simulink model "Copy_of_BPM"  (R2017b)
settings: Solver=FixedStepDiscrete  StartTime=0.0  StopTime=10.0  FixedStep=0.01  RelTol=1e-3  EnableMultiTasking=on
undefined symbols (not defined in the file): ASWTYPE_FALSE, CcBPM_KL30CHiVolt_mV, CcBPM_KL30CLoVolt_mV, CcBPM_KL30CTooHiVolt_mV, CcBPM_KL30CTooLoVolt_mV, CcBPM_KL30CVoltRtnDifVal_mV, CcBPM_KL30HiVolt_mV, CcBPM_KL30LoVolt_mV, CcBPM_KL30TooHiVolt_mV, CcBPM_KL30TooLoVolt_mV, CcBPM_KL30VoltRtnDifVal_mV, Enum_ISPBMULastPwrDown, Enum_ISPBMULastReset, Enum_ISPDiagComSt, Enum_ISPNetWkUpSt, Enum_MSMBMUState
libraries: AIWAYS_Powertrain_BMS_lib x15

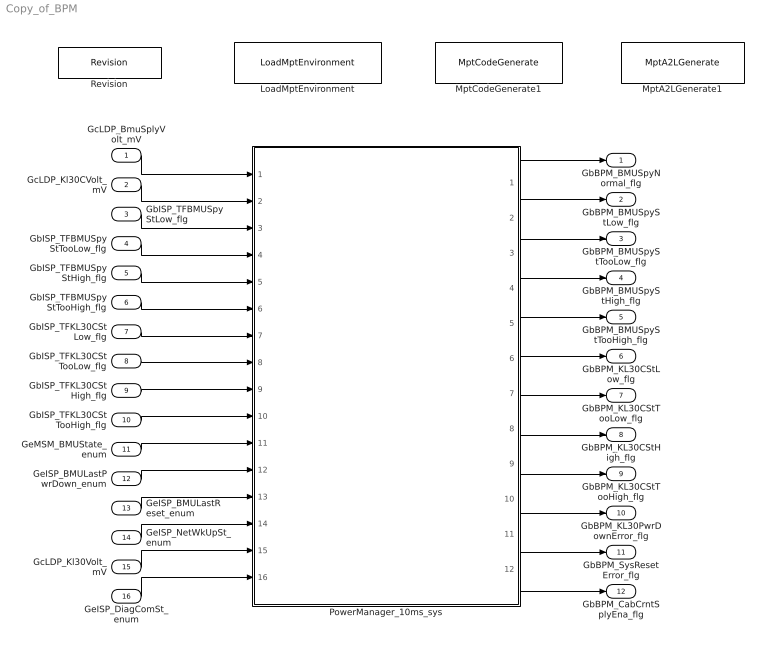
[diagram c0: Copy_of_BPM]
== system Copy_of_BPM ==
  GcLDP_BmuSplyVolt_mV : Inport
  GcLDP_Kl30CVolt_mV : Inport  Port=2
  GbISP_TFBMUSpyStLow_flg : Inport  Port=3
  GbISP_TFBMUSpyStTooLow_flg : Inport  Port=4
  GbISP_TFBMUSpyStHigh_flg : Inport  Port=5
  GbISP_TFBMUSpyStTooHigh_flg : Inport  Port=6
  GbISP_TFKL30CStLow_flg : Inport  Port=7
  GbISP_TFKL30CStTooLow_flg : Inport  Port=8
  GbISP_TFKL30CStHigh_flg : Inport  Port=9
  GbISP_TFKL30CStTooHigh_flg : Inport  Port=10
  GeMSM_BMUState_enum : Inport  Port=11
  GeISP_BMULastPwrDown_enum : Inport  Port=12
  GeISP_BMULastReset_enum : Inport  Port=13
  GeISP_NetWkUpSt_enum : Inport  Port=14
  GcLDP_Kl30Volt_mV : Inport  Port=15
  GeISP_DiagComSt_enum : Inport  Port=16
  LoadMptEnvironment : AIWAYS_Powertrain_BMS_lib/Config/LoadMptEnvironment  ProjectName=Comm  SuppierID=NewPlatformUAES
  MptA2LGenerate1 : AIWAYS_Powertrain_BMS_lib/Config/MptA2LGenerate  SystemSampleTime=-1
  MptCodeGenerate1 : AIWAYS_Powertrain_BMS_lib/Config/MptCodeGenerate  SystemSampleTime=-1
  PowerManager_10ms_sys : Subsystem
  Revision : AIWAYS_Powertrain_BMS_lib/Config/Revision  curVersion='M105C104'  newVersion='M105C104'
  GbBPM_BMUSpyNormal_flg : Outport
  GbBPM_BMUSpyStLow_flg : Outport  Port=2
  GbBPM_BMUSpyStTooLow_flg : Outport  Port=3
  GbBPM_BMUSpyStHigh_flg : Outport  Port=4
  GbBPM_BMUSpyStTooHigh_flg : Outport  Port=5
  GbBPM_KL30CStLow_flg : Outport  Port=6
  GbBPM_KL30CStTooLow_flg : Outport  Port=7
  GbBPM_KL30CStHigh_flg : Outport  Port=8
  GbBPM_KL30CStTooHigh_flg : Outport  Port=9
  GbBPM_KL30PwrDownError_flg : Outport  Port=10
  GbBPM_SysResetError_flg : Outport  Port=11
  GbBPM_CabCrntSplyEna_flg : Outport  Port=12
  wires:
  GcLDP_Kl30CVolt_mV/1 -> PowerManager_10ms_sys/2(GcLDP_Kl30CVolt_mV)
  GeISP_DiagComSt_enum/1 -> PowerManager_10ms_sys/16(GeISP_DiagComSt_enum)
  GbISP_TFBMUSpyStHigh_flg/1 -> PowerManager_10ms_sys/5(GbISP_TFBMUSpyStHigh_flg)
  GcLDP_BmuSplyVolt_mV/1 -> PowerManager_10ms_sys/1(GcLDP_BmuSplyVolt_mV)
  PowerManager_10ms_sys/2(GbBPM_BMUSpyStLow_flg) -> GbBPM_BMUSpyStLow_flg/1
  PowerManager_10ms_sys/8(GbBPM_KL30CStHigh_flg) -> GbBPM_KL30CStHigh_flg/1
  PowerManager_10ms_sys/4(GbBPM_BMUSpyStHigh_flg) -> GbBPM_BMUSpyStHigh_flg/1
  PowerManager_10ms_sys/1(GbBPM_BMUSpyNormal_flg) -> GbBPM_BMUSpyNormal_flg/1
  GbISP_TFKL30CStTooLow_flg/1 -> PowerManager_10ms_sys/8(GbISP_TFKL30CStTooLow_flg)
  GcLDP_Kl30Volt_mV/1 -> PowerManager_10ms_sys/15(GcLDP_Kl30Volt_mV)
  GeMSM_BMUState_enum/1 -> PowerManager_10ms_sys/11(GeMSM_BMUState_enum)
  GbISP_TFBMUSpyStTooLow_flg/1 -> PowerManager_10ms_sys/4(GbISP_TFBMUSpyStTooLow_flg)
  GbISP_TFKL30CStHigh_flg/1 -> PowerManager_10ms_sys/9(GbISP_TFKL30CStHigh_flg)
  PowerManager_10ms_sys/12(GbBPM_CabCrntSplyEna_flg) -> GbBPM_CabCrntSplyEna_flg/1
  PowerManager_10ms_sys/5(GbBPM_BMUSpyStTooHigh_flg) -> GbBPM_BMUSpyStTooHigh_flg/1
  GeISP_BMULastPwrDown_enum/1 -> PowerManager_10ms_sys/12(GeISP_BMULastPwrDown_enum)
  PowerManager_10ms_sys/3(GbBPM_BMUSpyStTooLow_flg) -> GbBPM_BMUSpyStTooLow_flg/1
  PowerManager_10ms_sys/6(GbBPM_KL30CStLow_flg) -> GbBPM_KL30CStLow_flg/1
  GbISP_TFBMUSpyStTooHigh_flg/1 -> PowerManager_10ms_sys/6(GbISP_TFBMUSpyStTooHigh_flg)
  PowerManager_10ms_sys/9(GbBPM_KL30CStTooHigh_flg) -> GbBPM_KL30CStTooHigh_flg/1
  GbISP_TFBMUSpyStLow_flg/1 -> PowerManager_10ms_sys/3(GbISP_TFBMUSpyStLow_flg)
  PowerManager_10ms_sys/11(GbBPM_SysResetError_flg) -> GbBPM_SysResetError_flg/1
  GeISP_NetWkUpSt_enum/1 -> PowerManager_10ms_sys/14(GeISP_NetWkUpSt_enum)
  GbISP_TFKL30CStLow_flg/1 -> PowerManager_10ms_sys/7(GbISP_TFKL30CStLow_flg)
  GbISP_TFKL30CStTooHigh_flg/1 -> PowerManager_10ms_sys/10(GbISP_TFKL30CStTooHigh_flg)
  PowerManager_10ms_sys/7(GbBPM_KL30CStTooLow_flg) -> GbBPM_KL30CStTooLow_flg/1
  GeISP_BMULastReset_enum/1 -> PowerManager_10ms_sys/13(GeISP_BMULastReset_enum)
  PowerManager_10ms_sys/10(GbBPM_KL30PwrDownError_flg) -> GbBPM_KL30PwrDownError_flg/1

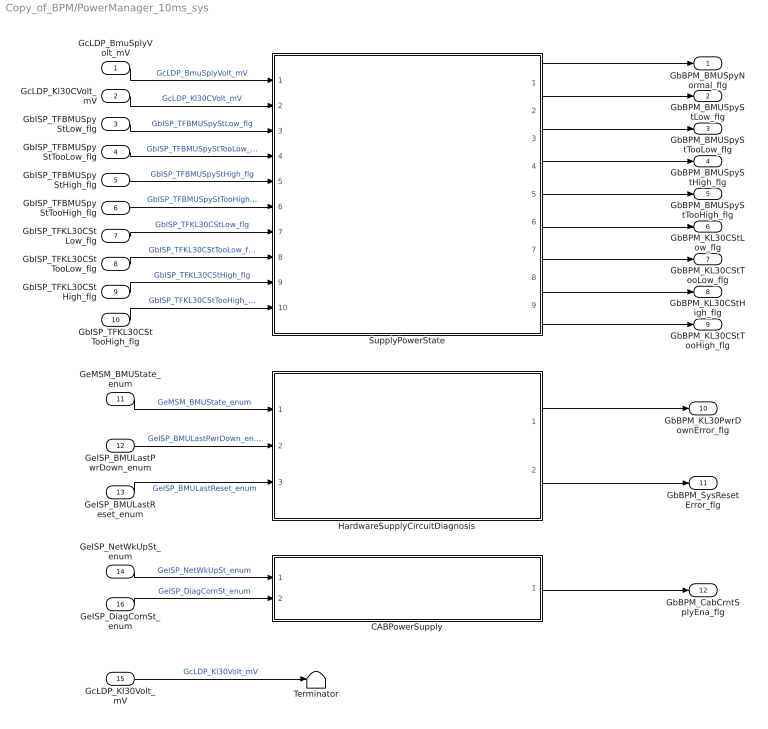
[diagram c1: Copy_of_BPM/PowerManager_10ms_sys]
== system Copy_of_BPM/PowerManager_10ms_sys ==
  GcLDP_BmuSplyVolt_mV : Inport
  GcLDP_Kl30CVolt_mV : Inport  Port=2
  GbISP_TFBMUSpyStLow_flg : Inport  Port=3
  GbISP_TFBMUSpyStTooLow_flg : Inport  Port=4
  GbISP_TFBMUSpyStHigh_flg : Inport  Port=5
  GbISP_TFBMUSpyStTooHigh_flg : Inport  Port=6
  GbISP_TFKL30CStLow_flg : Inport  Port=7
  GbISP_TFKL30CStTooLow_flg : Inport  Port=8
  GbISP_TFKL30CStHigh_flg : Inport  Port=9
  GbISP_TFKL30CStTooHigh_flg : Inport  Port=10
  GeMSM_BMUState_enum : Inport  Port=11
  GeISP_BMULastPwrDown_enum : Inport  Port=12
  GeISP_BMULastReset_enum : Inport  Port=13
  GeISP_NetWkUpSt_enum : Inport  Port=14
  GcLDP_Kl30Volt_mV : Inport  Port=15
  GeISP_DiagComSt_enum : Inport  Port=16
  CABPowerSupply : Subsystem
  HardwareSupplyCircuitDiagnosis : Subsystem
  SupplyPowerState : Subsystem
  Terminator : Terminator
  GbBPM_BMUSpyNormal_flg : Outport
  GbBPM_BMUSpyStLow_flg : Outport  Port=2
  GbBPM_BMUSpyStTooLow_flg : Outport  Port=3
  GbBPM_BMUSpyStHigh_flg : Outport  Port=4
  GbBPM_BMUSpyStTooHigh_flg : Outport  Port=5
  GbBPM_KL30CStLow_flg : Outport  Port=6
  GbBPM_KL30CStTooLow_flg : Outport  Port=7
  GbBPM_KL30CStHigh_flg : Outport  Port=8
  GbBPM_KL30CStTooHigh_flg : Outport  Port=9
  GbBPM_KL30PwrDownError_flg : Outport  Port=10
  GbBPM_SysResetError_flg : Outport  Port=11
  GbBPM_CabCrntSplyEna_flg : Outport  Port=12
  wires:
  GcLDP_BmuSplyVolt_mV/1 -> SupplyPowerState/1(GcLDP_BmuSplyVolt_mV)  "GcLDP_BmuSplyVolt_mV"
  GeMSM_BMUState_enum/1 -> HardwareSupplyCircuitDiagnosis/1(GeMSM_BMUState_enum)  "GeMSM_BMUState_enum"
  GeISP_BMULastPwrDown_enum/1 -> HardwareSupplyCircuitDiagnosis/2(GeISP_BMULastPwrDown_enum)  "GeISP_BMULastPwrDown_enum"
  GeISP_BMULastReset_enum/1 -> HardwareSupplyCircuitDiagnosis/3(GeISP_BMULastReset_enum)  "GeISP_BMULastReset_enum"
  SupplyPowerState/1(GbBPM_BMUSpyNormal_flg) -> GbBPM_BMUSpyNormal_flg/1
  HardwareSupplyCircuitDiagnosis/1(GbBPM_KL30PwrDownError_flg) -> GbBPM_KL30PwrDownError_flg/1
  HardwareSupplyCircuitDiagnosis/2(GbBPM_SysResetError_flg) -> GbBPM_SysResetError_flg/1
  SupplyPowerState/2(GbBPM_BMUSpyStLow_flg) -> GbBPM_BMUSpyStLow_flg/1
  SupplyPowerState/3(GbBPM_BMUSpyStTooLow_flg) -> GbBPM_BMUSpyStTooLow_flg/1
  SupplyPowerState/4(GbBPM_BMUSpyStHigh_flg) -> GbBPM_BMUSpyStHigh_flg/1
  SupplyPowerState/5(GbBPM_BMUSpyStTooHigh_flg) -> GbBPM_BMUSpyStTooHigh_flg/1
  CABPowerSupply/1(GbBPM_CabCrntSplyEna_flg) -> GbBPM_CabCrntSplyEna_flg/1
  GcLDP_Kl30Volt_mV/1 -> Terminator/1  "GcLDP_Kl30Volt_mV"
  GeISP_NetWkUpSt_enum/1 -> CABPowerSupply/1(GeISP_NetWkUpSt_enum)  "GeISP_NetWkUpSt_enum"
  GcLDP_Kl30CVolt_mV/1 -> SupplyPowerState/2(GcLDP_Kl30CVolt_mV)  "GcLDP_Kl30CVolt_mV"
  SupplyPowerState/6(GbBPM_KL30CStLow_flg) -> GbBPM_KL30CStLow_flg/1
  SupplyPowerState/7(GbBPM_KL30CStTooLow_flg) -> GbBPM_KL30CStTooLow_flg/1
  SupplyPowerState/8(GbBPM_KL30CStHigh_flg) -> GbBPM_KL30CStHigh_flg/1
  SupplyPowerState/9(GbBPM_KL30CStTooHigh_flg) -> GbBPM_KL30CStTooHigh_flg/1
  GbISP_TFBMUSpyStLow_flg/1 -> SupplyPowerState/3(GbISP_TFBMUSpyStLow_flg)  "GbISP_TFBMUSpyStLow_flg"
  GbISP_TFBMUSpyStTooLow_flg/1 -> SupplyPowerState/4(GbISP_TFBMUSpyStTooLow_flg)  "GbISP_TFBMUSpyStTooLow_flg"
  GbISP_TFBMUSpyStHigh_flg/1 -> SupplyPowerState/5(GbISP_TFBMUSpyStHigh_flg)  "GbISP_TFBMUSpyStHigh_flg"
  GbISP_TFBMUSpyStTooHigh_flg/1 -> SupplyPowerState/6(GbISP_TFBMUSpyStTooHigh_flg)  "GbISP_TFBMUSpyStTooHigh_flg"
  GbISP_TFKL30CStLow_flg/1 -> SupplyPowerState/7(GbISP_TFKL30CStLow_flg)  "GbISP_TFKL30CStLow_flg"
  GbISP_TFKL30CStTooLow_flg/1 -> SupplyPowerState/8(GbISP_TFKL30CStTooLow_flg)  "GbISP_TFKL30CStTooLow_flg"
  GbISP_TFKL30CStHigh_flg/1 -> SupplyPowerState/9(GbISP_TFKL30CStHigh_flg)  "GbISP_TFKL30CStHigh_flg"
  GbISP_TFKL30CStTooHigh_flg/1 -> SupplyPowerState/10(GbISP_TFKL30CStTooHigh_flg)  "GbISP_TFKL30CStTooHigh_flg"
  GeISP_DiagComSt_enum/1 -> CABPowerSupply/2(GeISP_DiagComSt_enum)  "GeISP_DiagComSt_enum"

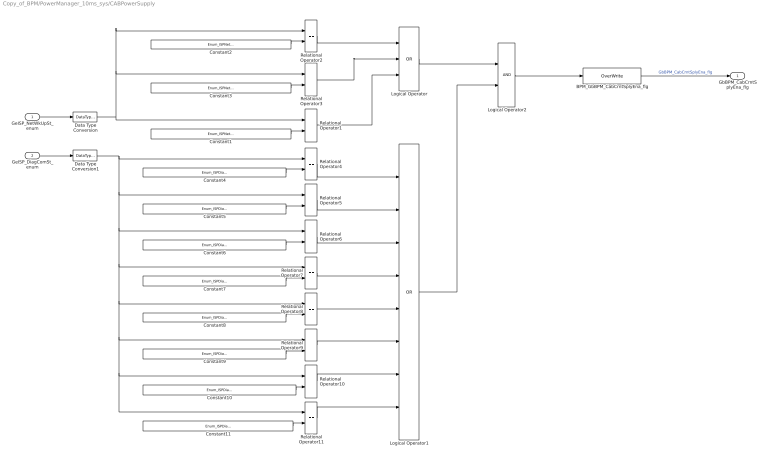
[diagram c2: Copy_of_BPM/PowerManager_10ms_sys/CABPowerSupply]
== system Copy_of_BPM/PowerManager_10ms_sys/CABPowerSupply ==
  GeISP_NetWkUpSt_enum : Inport
  GeISP_DiagComSt_enum : Inport  Port=2
  BPM_GbBPM_CabCrntSplyEna_flg : AIWAYS_Powertrain_BMS_lib/Signals/OverWrite  OverWrite_Value=CbBPM_CabCrntSplyEnaOvr_flg  OverWrite_flag=CbBPM_CabCrntSplyEnaOvrSwt_flg
  Constant1 : Constant  Value=Enum_ISPNetWkUpSt.Enum_ISPNetWkUpSt_ReadySleep
  Constant10 : Constant  Value=Enum_ISPDiagComSt.Enum_ISPDiagComSt_NMAppMsgRxEnTxEn
  Constant11 : Constant  Value=Enum_ISPDiagComSt.Enum_ISPDiagComSt_NMAppMsgRxDsTxEn
  Constant2 : Constant  Value=Enum_ISPNetWkUpSt.Enum_ISPNetWkUpSt_NormalOperation
  Constant3 : Constant  Value=Enum_ISPNetWkUpSt.Enum_ISPNetWkUpSt_RepeatMessage
  Constant4 : Constant  Value=Enum_ISPDiagComSt.Enum_ISPDiagComSt_AppMsgRxEnTxEn
  Constant5 : Constant  Value=Enum_ISPDiagComSt.Enum_ISPDiagComSt_AppMsgRxDsTxEn
  Constant6 : Constant  Value=Enum_ISPDiagComSt.Enum_ISPDiagComSt_NMMsgRxEnTxEn
  Constant7 : Constant  Value=Enum_ISPDiagComSt.Enum_ISPDiagComSt_NMMsgRxEnTxDs
  Constant8 : Constant  Value=Enum_ISPDiagComSt.Enum_ISPDiagComSt_NMMsgRxDsTxEn
  Constant9 : Constant  Value=Enum_ISPDiagComSt.Enum_ISPDiagComSt_NMMsgRxDsTxDs
  Data Type Conversion : DataTypeConversion
  Data Type Conversion1 : DataTypeConversion
  Logical Operator : Logic  Operator=OR  Inputs=3  AllPortsSameDT=off  OutDataTypeStr=boolean
  Logical Operator1 : Logic  Operator=OR  Inputs=8  AllPortsSameDT=off  OutDataTypeStr=boolean
  Logical Operator2 : Logic  AllPortsSameDT=off  OutDataTypeStr=boolean
  Relational Operator{1..11} (11 alike) : RelationalOperator  Operator===  OutDataTypeStr=boolean
  GbBPM_CabCrntSplyEna_flg : Outport
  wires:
  BPM_GbBPM_CabCrntSplyEna_flg/1 -> GbBPM_CabCrntSplyEna_flg/1  "GbBPM_CabCrntSplyEna_flg"
  Relational Operator2/1 -> Logical Operator/1
  Data Type Conversion/1 -> Relational Operator2/1, Relational Operator3/1, Relational Operator1/1
  GeISP_NetWkUpSt_enum/1 -> Data Type Conversion/1
  Constant3/1 -> Relational Operator3/2
  Relational Operator3/1 -> Logical Operator/2
  Constant2/1 -> Relational Operator2/2
  Constant1/1 -> Relational Operator1/2
  Relational Operator1/1 -> Logical Operator/3
  GeISP_DiagComSt_enum/1 -> Data Type Conversion1/1
  Relational Operator4/1 -> Logical Operator1/1
  Logical Operator/1 -> Logical Operator2/1
  Logical Operator2/1 -> BPM_GbBPM_CabCrntSplyEna_flg/1
  Logical Operator1/1 -> Logical Operator2/2
  Constant4/1 -> Relational Operator4/2
  Relational Operator5/1 -> Logical Operator1/2
  Constant5/1 -> Relational Operator5/2
  Relational Operator6/1 -> Logical Operator1/3
  Constant6/1 -> Relational Operator6/2
  Relational Operator7/1 -> Logical Operator1/4
  Constant7/1 -> Relational Operator7/2
  Relational Operator8/1 -> Logical Operator1/5
  Constant8/1 -> Relational Operator8/2
  Relational Operator9/1 -> Logical Operator1/6
  Constant9/1 -> Relational Operator9/2
  Relational Operator10/1 -> Logical Operator1/7
  Constant10/1 -> Relational Operator10/2
  Relational Operator11/1 -> Logical Operator1/8
  Data Type Conversion1/1 -> Relational Operator11/1, Relational Operator10/1, Relational Operator9/1, Relational Operator8/1, Relational Operator7/1, Relational Operator6/1, Relational Operator5/1, Relational Operator4/1
  Constant11/1 -> Relational Operator11/2

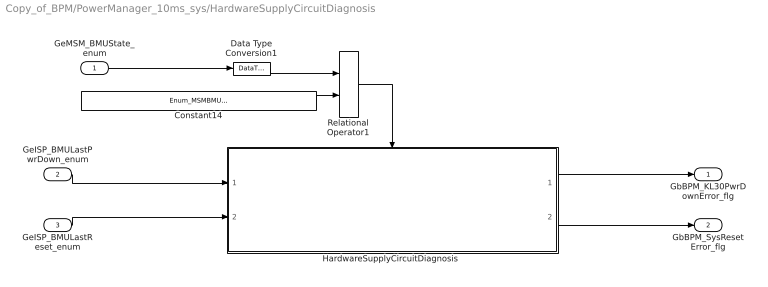
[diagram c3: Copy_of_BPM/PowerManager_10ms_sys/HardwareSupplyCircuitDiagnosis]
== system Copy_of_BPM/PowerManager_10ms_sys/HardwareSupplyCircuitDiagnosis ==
  GeMSM_BMUState_enum : Inport
  GeISP_BMULastPwrDown_enum : Inport  Port=2
  GeISP_BMULastReset_enum : Inport  Port=3
  Constant14 : Constant  Value=Enum_MSMBMUState.Enum_MSMBMUState_Standby
  Data Type Conversion1 : DataTypeConversion
  "HardwareSupplyCircuitDiagnosis " : Subsystem  TreatAsAtomicUnit=on
  Relational Operator1 : RelationalOperator  Operator===  OutDataTypeStr=boolean
  GbBPM_KL30PwrDownError_flg : Outport
  GbBPM_SysResetError_flg : Outport  Port=2
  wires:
  Relational Operator1/1 -> "HardwareSupplyCircuitDiagnosis "/Enable
  Data Type Conversion1/1 -> Relational Operator1/1
  "HardwareSupplyCircuitDiagnosis "/2(GbBPM_SysResetError_flg) -> GbBPM_SysResetError_flg/1
  Constant14/1 -> Relational Operator1/2
  "HardwareSupplyCircuitDiagnosis "/1(GbBPM_KL30PwrDownError_flg) -> GbBPM_KL30PwrDownError_flg/1
  GeISP_BMULastPwrDown_enum/1 -> "HardwareSupplyCircuitDiagnosis "/1(GeISP_BMULastPwrDown_enum)
  GeMSM_BMUState_enum/1 -> Data Type Conversion1/1
  GeISP_BMULastReset_enum/1 -> "HardwareSupplyCircuitDiagnosis "/2(GeISP_BMULastReset_enum)

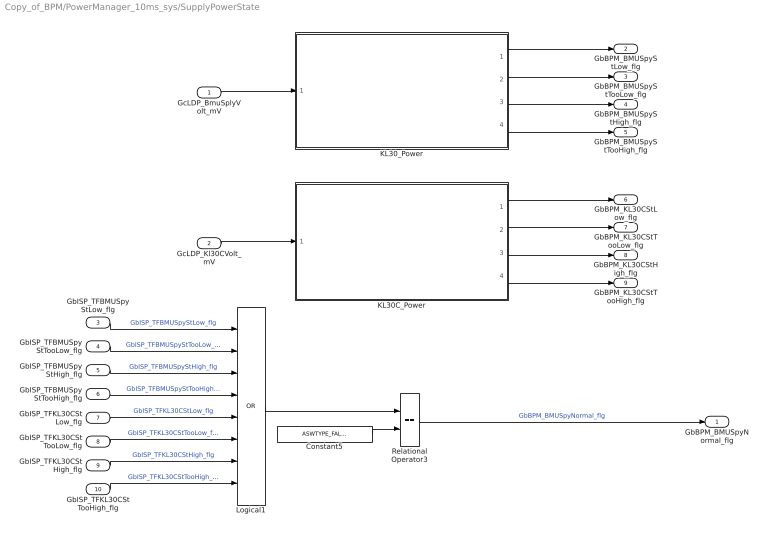
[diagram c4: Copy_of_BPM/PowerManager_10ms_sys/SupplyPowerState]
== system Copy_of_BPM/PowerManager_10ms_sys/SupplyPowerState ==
  GcLDP_BmuSplyVolt_mV : Inport
  GcLDP_Kl30CVolt_mV : Inport  Port=2
  GbISP_TFBMUSpyStLow_flg : Inport  Port=3
  GbISP_TFBMUSpyStTooLow_flg : Inport  Port=4
  GbISP_TFBMUSpyStHigh_flg : Inport  Port=5
  GbISP_TFBMUSpyStTooHigh_flg : Inport  Port=6
  GbISP_TFKL30CStLow_flg : Inport  Port=7
  GbISP_TFKL30CStTooLow_flg : Inport  Port=8
  GbISP_TFKL30CStHigh_flg : Inport  Port=9
  GbISP_TFKL30CStTooHigh_flg : Inport  Port=10
  Constant5 : Constant  Value=ASWTYPE_FALSE
  KL30C_Power : Subsystem
  KL30_Power : Subsystem
  Logical1 : Logic  Operator=OR  Inputs=8  OutDataTypeStr=boolean
  Relational Operator3 : RelationalOperator  Operator===  OutDataTypeStr=boolean
  GbBPM_BMUSpyNormal_flg : Outport
  GbBPM_BMUSpyStLow_flg : Outport  Port=2
  GbBPM_BMUSpyStTooLow_flg : Outport  Port=3
  GbBPM_BMUSpyStHigh_flg : Outport  Port=4
  GbBPM_BMUSpyStTooHigh_flg : Outport  Port=5
  GbBPM_KL30CStLow_flg : Outport  Port=6
  GbBPM_KL30CStTooLow_flg : Outport  Port=7
  GbBPM_KL30CStHigh_flg : Outport  Port=8
  GbBPM_KL30CStTooHigh_flg : Outport  Port=9
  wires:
  Relational Operator3/1 -> GbBPM_BMUSpyNormal_flg/1  "GbBPM_BMUSpyNormal_flg"
  GcLDP_BmuSplyVolt_mV/1 -> KL30_Power/1(GcLDP_BmuSplyVolt_mV)
  KL30_Power/1(GbBPM_BMUSpyStLow_flg) -> GbBPM_BMUSpyStLow_flg/1
  KL30_Power/2(GbBPM_BMUSpyStTooLow_flg) -> GbBPM_BMUSpyStTooLow_flg/1
  KL30_Power/3(GbBPM_BMUSpyStHigh_flg) -> GbBPM_BMUSpyStHigh_flg/1
  KL30_Power/4(GbBPM_BMUSpyStTooHigh_flg) -> GbBPM_BMUSpyStTooHigh_flg/1
  GcLDP_Kl30CVolt_mV/1 -> KL30C_Power/1(GcLDP_Kl30CVolt_mV)
  KL30C_Power/1(GbBPM_KL30CStLow_flg) -> GbBPM_KL30CStLow_flg/1
  KL30C_Power/2(GbBPM_KL30CStTooLow_flg) -> GbBPM_KL30CStTooLow_flg/1
  KL30C_Power/3(GbBPM_KL30CStHigh_flg) -> GbBPM_KL30CStHigh_flg/1
  KL30C_Power/4(GbBPM_KL30CStTooHigh_flg) -> GbBPM_KL30CStTooHigh_flg/1
  GbISP_TFBMUSpyStTooLow_flg/1 -> Logical1/2  "GbISP_TFBMUSpyStTooLow_flg"
  GbISP_TFBMUSpyStHigh_flg/1 -> Logical1/3  "GbISP_TFBMUSpyStHigh_flg"
  GbISP_TFBMUSpyStTooHigh_flg/1 -> Logical1/4  "GbISP_TFBMUSpyStTooHigh_flg"
  GbISP_TFKL30CStLow_flg/1 -> Logical1/5  "GbISP_TFKL30CStLow_flg"
  GbISP_TFKL30CStTooLow_flg/1 -> Logical1/6  "GbISP_TFKL30CStTooLow_flg"
  GbISP_TFKL30CStHigh_flg/1 -> Logical1/7  "GbISP_TFKL30CStHigh_flg"
  GbISP_TFKL30CStTooHigh_flg/1 -> Logical1/8  "GbISP_TFKL30CStTooHigh_flg"
  GbISP_TFBMUSpyStLow_flg/1 -> Logical1/1  "GbISP_TFBMUSpyStLow_flg"
  Logical1/1 -> Relational Operator3/1
  Constant5/1 -> Relational Operator3/2

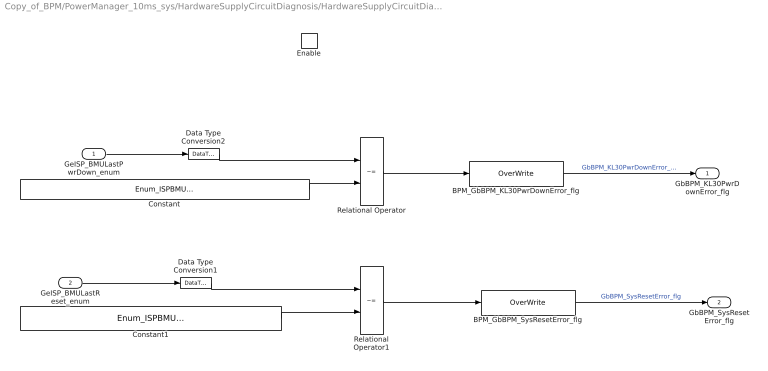
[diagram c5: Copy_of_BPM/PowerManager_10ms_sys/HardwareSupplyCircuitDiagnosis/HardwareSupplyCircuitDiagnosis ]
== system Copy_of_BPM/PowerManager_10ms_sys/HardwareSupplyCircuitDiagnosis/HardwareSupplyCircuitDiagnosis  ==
  GeISP_BMULastPwrDown_enum : Inport
  GeISP_BMULastReset_enum : Inport  Port=2
  Enable : EnablePort  StatesWhenEnabling=reset
  BPM_GbBPM_KL30PwrDownError_flg : AIWAYS_Powertrain_BMS_lib/Signals/OverWrite  OverWrite_Value=CbBPM_KL30PwrDownErrorOvr_flg  OverWrite_flag=CbBPM_KL30PwrDownErrorOvrSwt_flg
  BPM_GbBPM_SysResetError_flg : AIWAYS_Powertrain_BMS_lib/Signals/OverWrite  OverWrite_Value=CbBPM_SysResetErrorOvr_flg  OverWrite_flag=CbBPM_SysResetErrorOvrSwt_flg
  Constant : Constant  Value=Enum_ISPBMULastPwrDown.Enum_ISPBMULastPwrDown_PwrSpyConnect
  Constant1 : Constant  Value=Enum_ISPBMULastReset.Enum_ISPBMULastReset_NoReset
  Data Type Conversion1 : DataTypeConversion
  Data Type Conversion2 : DataTypeConversion
  Relational Operator : RelationalOperator  Operator=~=  OutDataTypeStr=boolean
  Relational Operator1 : RelationalOperator  Operator=~=  OutDataTypeStr=boolean
  GbBPM_KL30PwrDownError_flg : Outport
  GbBPM_SysResetError_flg : Outport  Port=2
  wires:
  BPM_GbBPM_KL30PwrDownError_flg/1 -> GbBPM_KL30PwrDownError_flg/1  "GbBPM_KL30PwrDownError_flg"
  BPM_GbBPM_SysResetError_flg/1 -> GbBPM_SysResetError_flg/1  "GbBPM_SysResetError_flg"
  Constant/1 -> Relational Operator/2
  Constant1/1 -> Relational Operator1/2
  GeISP_BMULastPwrDown_enum/1 -> Data Type Conversion2/1
  Data Type Conversion2/1 -> Relational Operator/1
  Relational Operator/1 -> BPM_GbBPM_KL30PwrDownError_flg/1
  Data Type Conversion1/1 -> Relational Operator1/1
  GeISP_BMULastReset_enum/1 -> Data Type Conversion1/1
  Relational Operator1/1 -> BPM_GbBPM_SysResetError_flg/1

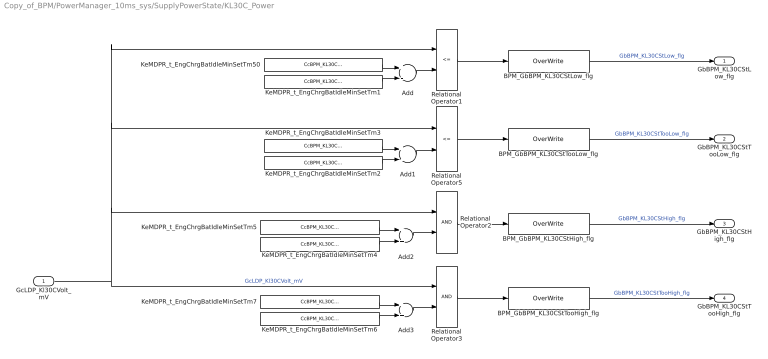
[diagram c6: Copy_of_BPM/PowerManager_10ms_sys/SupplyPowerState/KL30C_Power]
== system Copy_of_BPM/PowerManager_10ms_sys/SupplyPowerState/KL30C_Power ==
  GcLDP_Kl30CVolt_mV : Inport
  Add : Sum  Inputs=+-  OutDataTypeStr=Inherit: Inherit via back propagation
  Add1 : Sum  Inputs=+-  OutDataTypeStr=Inherit: Inherit via back propagation
  Add2 : Sum  OutDataTypeStr=Inherit: Inherit via back propagation
  Add3 : Sum
  BPM_GbBPM_KL30CStHigh_flg : AIWAYS_Powertrain_BMS_lib/Signals/OverWrite  OverWrite_Value=CbBPM_KL30CStHighOvr_flg  OverWrite_flag=CbBPM_KL30CStHighOvrSwt_flg
  BPM_GbBPM_KL30CStLow_flg : AIWAYS_Powertrain_BMS_lib/Signals/OverWrite  OverWrite_Value=CbBPM_KL30CStLowOvr_flg  OverWrite_flag=CbBPM_KL30CStLowOvrSwt_flg
  BPM_GbBPM_KL30CStTooHigh_flg : AIWAYS_Powertrain_BMS_lib/Signals/OverWrite  OverWrite_Value=CbBPM_KL30CStTooHighOvr_flg  OverWrite_flag=CbBPM_KL30CStTooHighOvrSwt_flg
  BPM_GbBPM_KL30CStTooLow_flg : AIWAYS_Powertrain_BMS_lib/Signals/OverWrite  OverWrite_Value=CbBPM_KL30CStTooLowOvr_flg  OverWrite_flag=CbBPM_KL30CStTooLowOvrSwt_flg
  KeMDPR_t_EngChrgBatIdleMinSetTm{1..2,4,6} (4 alike) : Constant  Value=CcBPM_KL30CVoltRtnDifVal_mV
  KeMDPR_t_EngChrgBatIdleMinSetTm3 : Constant  Value=CcBPM_KL30CTooLoVolt_mV
  KeMDPR_t_EngChrgBatIdleMinSetTm5 : Constant  Value=CcBPM_KL30CHiVolt_mV
  KeMDPR_t_EngChrgBatIdleMinSetTm50 : Constant  Value=CcBPM_KL30CLoVolt_mV
  KeMDPR_t_EngChrgBatIdleMinSetTm7 : Constant  Value=CcBPM_KL30CTooHiVolt_mV
  Relational Operator1 : RelationalOperator  Operator=<=  OutDataTypeStr=boolean
  Relational Operator2 : RelationalOperator  OutDataTypeStr=boolean
  Relational Operator3 : RelationalOperator  OutDataTypeStr=boolean
  Relational Operator5 : RelationalOperator  Operator=<=  OutDataTypeStr=boolean
  GbBPM_KL30CStLow_flg : Outport
  GbBPM_KL30CStTooLow_flg : Outport  Port=2
  GbBPM_KL30CStHigh_flg : Outport  Port=3
  GbBPM_KL30CStTooHigh_flg : Outport  Port=4
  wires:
  KeMDPR_t_EngChrgBatIdleMinSetTm7/1 -> Add3/1
  Add3/1 -> Relational Operator3/2
  KeMDPR_t_EngChrgBatIdleMinSetTm6/1 -> Add3/2
  Add2/1 -> Relational Operator2/2
  KeMDPR_t_EngChrgBatIdleMinSetTm5/1 -> Add2/1
  KeMDPR_t_EngChrgBatIdleMinSetTm4/1 -> Add2/2
  KeMDPR_t_EngChrgBatIdleMinSetTm2/1 -> Add1/2
  KeMDPR_t_EngChrgBatIdleMinSetTm3/1 -> Add1/1
  Add1/1 -> Relational Operator5/2
  Add/1 -> Relational Operator1/2
  KeMDPR_t_EngChrgBatIdleMinSetTm1/1 -> Add/2
  KeMDPR_t_EngChrgBatIdleMinSetTm50/1 -> Add/1
  GcLDP_Kl30CVolt_mV/1 -> Relational Operator3/1, Relational Operator2/1, Relational Operator5/1, Relational Operator1/1  "GcLDP_Kl30CVolt_mV"
  Relational Operator1/1 -> BPM_GbBPM_KL30CStLow_flg/1
  Relational Operator3/1 -> BPM_GbBPM_KL30CStTooHigh_flg/1
  Relational Operator2/1 -> BPM_GbBPM_KL30CStHigh_flg/1
  Relational Operator5/1 -> BPM_GbBPM_KL30CStTooLow_flg/1
  BPM_GbBPM_KL30CStLow_flg/1 -> GbBPM_KL30CStLow_flg/1  "GbBPM_KL30CStLow_flg"
  BPM_GbBPM_KL30CStTooLow_flg/1 -> GbBPM_KL30CStTooLow_flg/1  "GbBPM_KL30CStTooLow_flg"
  BPM_GbBPM_KL30CStHigh_flg/1 -> GbBPM_KL30CStHigh_flg/1  "GbBPM_KL30CStHigh_flg"
  BPM_GbBPM_KL30CStTooHigh_flg/1 -> GbBPM_KL30CStTooHigh_flg/1  "GbBPM_KL30CStTooHigh_flg"

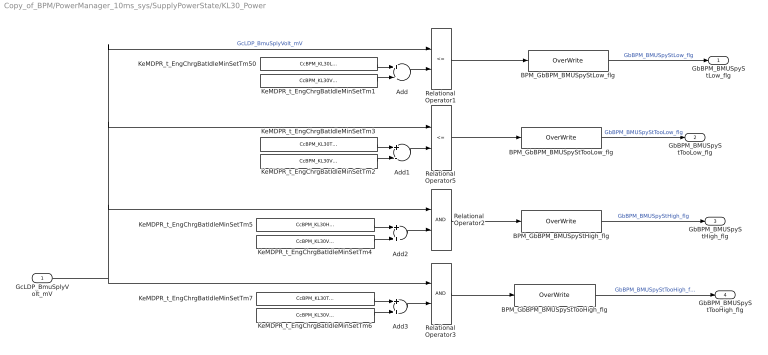
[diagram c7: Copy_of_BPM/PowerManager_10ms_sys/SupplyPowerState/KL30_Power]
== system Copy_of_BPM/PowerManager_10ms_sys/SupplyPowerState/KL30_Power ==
  GcLDP_BmuSplyVolt_mV : Inport
  Add : Sum  Inputs=+-  OutDataTypeStr=Inherit: Inherit via back propagation
  Add1 : Sum  Inputs=+-  OutDataTypeStr=Inherit: Inherit via back propagation
  Add2 : Sum  OutDataTypeStr=Inherit: Inherit via back propagation
  Add3 : Sum
  BPM_GbBPM_BMUSpyStHigh_flg : AIWAYS_Powertrain_BMS_lib/Signals/OverWrite  OverWrite_Value=CbBPM_BMUSpyStHighOvr_flg  OverWrite_flag=CbBPM_BMUSpyStHighOvrSwt_flg
  BPM_GbBPM_BMUSpyStLow_flg : AIWAYS_Powertrain_BMS_lib/Signals/OverWrite  OverWrite_Value=CbBPM_BMUSpyStLowOvr_flg  OverWrite_flag=CbBPM_BMUSpyStLowOvrSwt_flg
  BPM_GbBPM_BMUSpyStTooHigh_flg : AIWAYS_Powertrain_BMS_lib/Signals/OverWrite  OverWrite_Value=CbBPM_BMUSpyStTooHighOvr_flg  OverWrite_flag=CbBPM_BMUSpyStTooHighOvrSwt_flg
  BPM_GbBPM_BMUSpyStTooLow_flg : AIWAYS_Powertrain_BMS_lib/Signals/OverWrite  OverWrite_Value=CbBPM_BMUSpyStTooLowOvr_flg  OverWrite_flag=CbBPM_BMUSpyStTooLowOvrSwt_flg
  KeMDPR_t_EngChrgBatIdleMinSetTm{1..2,4,6} (4 alike) : Constant  Value=CcBPM_KL30VoltRtnDifVal_mV
  KeMDPR_t_EngChrgBatIdleMinSetTm3 : Constant  Value=CcBPM_KL30TooLoVolt_mV
  KeMDPR_t_EngChrgBatIdleMinSetTm5 : Constant  Value=CcBPM_KL30HiVolt_mV
  KeMDPR_t_EngChrgBatIdleMinSetTm50 : Constant  Value=CcBPM_KL30LoVolt_mV
  KeMDPR_t_EngChrgBatIdleMinSetTm7 : Constant  Value=CcBPM_KL30TooHiVolt_mV
  Relational Operator1 : RelationalOperator  Operator=<=  OutDataTypeStr=boolean
  Relational Operator2 : RelationalOperator  OutDataTypeStr=boolean
  Relational Operator3 : RelationalOperator  OutDataTypeStr=boolean
  Relational Operator5 : RelationalOperator  Operator=<=  OutDataTypeStr=boolean
  GbBPM_BMUSpyStLow_flg : Outport
  GbBPM_BMUSpyStTooLow_flg : Outport  Port=2
  GbBPM_BMUSpyStHigh_flg : Outport  Port=3
  GbBPM_BMUSpyStTooHigh_flg : Outport  Port=4
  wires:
  GcLDP_BmuSplyVolt_mV/1 -> Relational Operator1/1, Relational Operator5/1, Relational Operator2/1, Relational Operator3/1  "GcLDP_BmuSplyVolt_mV"
  BPM_GbBPM_BMUSpyStLow_flg/1 -> GbBPM_BMUSpyStLow_flg/1  "GbBPM_BMUSpyStLow_flg"
  BPM_GbBPM_BMUSpyStTooLow_flg/1 -> GbBPM_BMUSpyStTooLow_flg/1  "GbBPM_BMUSpyStTooLow_flg"
  BPM_GbBPM_BMUSpyStHigh_flg/1 -> GbBPM_BMUSpyStHigh_flg/1  "GbBPM_BMUSpyStHigh_flg"
  BPM_GbBPM_BMUSpyStTooHigh_flg/1 -> GbBPM_BMUSpyStTooHigh_flg/1  "GbBPM_BMUSpyStTooHigh_flg"
  KeMDPR_t_EngChrgBatIdleMinSetTm50/1 -> Add/1
  KeMDPR_t_EngChrgBatIdleMinSetTm1/1 -> Add/2
  Add/1 -> Relational Operator1/2
  Add1/1 -> Relational Operator5/2
  KeMDPR_t_EngChrgBatIdleMinSetTm3/1 -> Add1/1
  KeMDPR_t_EngChrgBatIdleMinSetTm2/1 -> Add1/2
  KeMDPR_t_EngChrgBatIdleMinSetTm4/1 -> Add2/2
  KeMDPR_t_EngChrgBatIdleMinSetTm5/1 -> Add2/1
  Add2/1 -> Relational Operator2/2
  KeMDPR_t_EngChrgBatIdleMinSetTm6/1 -> Add3/2
  Add3/1 -> Relational Operator3/2
  KeMDPR_t_EngChrgBatIdleMinSetTm7/1 -> Add3/1
  Relational Operator3/1 -> BPM_GbBPM_BMUSpyStTooHigh_flg/1
  Relational Operator2/1 -> BPM_GbBPM_BMUSpyStHigh_flg/1
  Relational Operator5/1 -> BPM_GbBPM_BMUSpyStTooLow_flg/1
  Relational Operator1/1 -> BPM_GbBPM_BMUSpyStLow_flg/1
